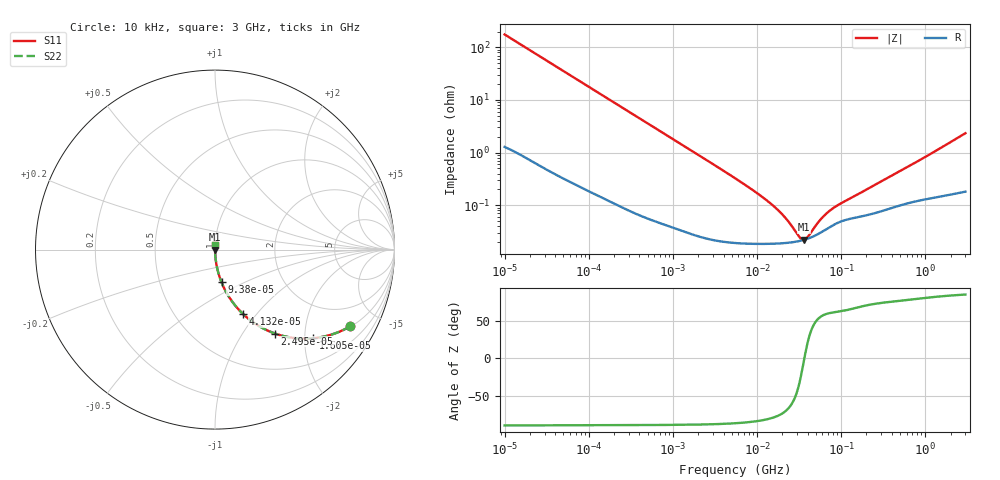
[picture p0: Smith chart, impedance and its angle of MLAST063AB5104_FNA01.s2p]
! MLAST063AB5104_FNA01  S-PARAMETER MODEL  ( Standard Model )
! Model Generated by TAIYO YUDEN Corporation (http://www.ty-top.com)
! Version 1.0
! TAIYO YUDEN Control No. 220601
! Copyright(c) 2014 TAIYO YUDEN CO.,LTD. All Rights Reserved.
! Product Description (link to TY-COMPAS)
! https://ds.yuden.co.jp/TYCOMPAS/or/detail?pn=MLAST063AB5104KFNA01&u=M
! Products Name : Multilayer Ceramic Capacitors
! Characteristics :
!  Capacitance : 0.1 [uF] , Rated Voltage : 25 [V] , TCC : X5R
!  Case Size : 0.6 x 0.3 / 0.024 x 0.012 [mm/inch] , Thickness : 0.3 / 0.012 [mm/inch]
!  (Conditions: Temperature = 25 [degC] , DC Bias Voltage = 0 [V])
! External Node Assignments :
!  1  o---| |---o  2
! GND o---------o GND
! Frequency Range : 10kHz  -  3GHz  [ 401 STEP ]
# MHZ S RI R 50
! Freq[MHz].  S11 Real  S11 Imag  S21 Real  S21 Imag  S12 Real  S12 Imag  S22 Real  S22 Imag
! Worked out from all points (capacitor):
!   401 points, 10 kHz to 3 GHz, reference 50 ohm
!   read as one part in series: C = 90.4 nF near 10.65 kHz
!   lowest |Z| = 22 mohm at 36.32 MHz (marker M1)
!   series resonance near 36.53 MHz, so ESL is about 210 pH
!   S11 on the Smith chart (normalised r, x): 10 kHz: 1.03, -3.51; 16.05 kHz: 1.02, -2.20; 24.95 kHz: 1.01, -1.42; 41.32 kHz: 1.01, -0.86; 93.8 kHz: 1.00, -0.38; 3 GHz: 1.00, +0.05
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0.01  0.7538 -0.4271  0.2462 0.4271  0.2462 0.4271  0.7538 -0.4271
0.016047  0.5463 -0.4939  0.4537 0.4939  0.4537 0.4939  0.5463 -0.4939
0.024951  0.3352 -0.4679  0.6648 0.4679  0.6648 0.4679  0.3352 -0.4679
0.041322  0.1574 -0.3598  0.8426 0.3598  0.8426 0.3598  0.1574 -0.3598
0.056638  0.0915 -0.2837  0.9085 0.2837  0.9085 0.2837  0.0915 -0.2837
0.082683  0.046 -0.2047  0.954 0.2047  0.954 0.2047  0.046 -0.2047
0.093797  0.0365 -0.1824  0.9635 0.1824  0.9635 0.1824  0.0365 -0.1824
0.219733  0.00756 -0.0807  0.9924 0.0807  0.9924 0.0807  0.00756 -0.0807
0.683653  0.00116 -0.0263  0.9988 0.0263  0.9988 0.0263  0.00116 -0.0263
5.477226  0.000202 -0.00326  0.9998 0.00326  0.9998 0.00326  0.000202 -0.00326
10.29003  0.000187 -0.00164  0.9998 0.00164  0.9998 0.00164  0.000187 -0.00164
15.99985  0.000186 -0.000924  0.9998 0.000924  0.9998 0.000924  0.000186 -0.000924
22.63272  0.000193 -0.000498  0.9998 0.000498  0.9998 0.000498  0.000193 -0.000498
32.0153  0.000209 -0.000132  0.9998 0.000132  0.9998 0.000132  0.000209 -0.000132
34.09912  0.000214 -6.87e-05  0.9998 6.87e-05  0.9998 6.87e-05  0.000214 -6.87e-05
36.31858  0.00022 -5.6e-06  0.9998 5.6e-06  0.9998 5.6e-06  0.00022 -5.6e-06
39.92153  0.000231 8.87e-05  0.9998 -8.87e-05  0.9998 -8.87e-05  0.000231 8.87e-05
45.28751  0.000249 0.000214  0.9998 -0.000214  0.9998 -0.000214  0.000249 0.000214
60.14696  0.000317 0.000497  0.9997 -0.000497  0.9997 -0.000497  0.000317 0.000497
79.88199  0.000416 0.000767  0.9996 -0.000767  0.9996 -0.000767  0.000416 0.000767
374.4521  0.000867 0.00335  0.9991 -0.00335  0.9991 -0.00335  0.000867 0.00335
3000  0.00235 0.0232  0.9977 -0.0232  0.9977 -0.0232  0.00235 0.0232
